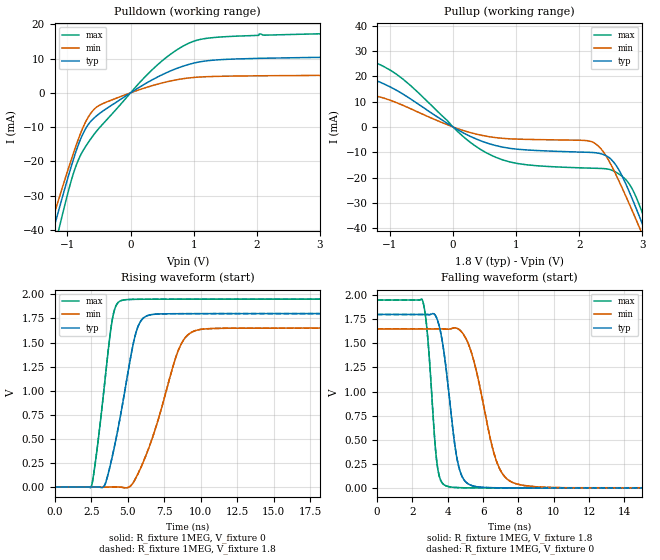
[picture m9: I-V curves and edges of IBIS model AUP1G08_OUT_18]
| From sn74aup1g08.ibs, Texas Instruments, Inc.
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[Model]   AUP1G08_OUT_18
Model_type  Output
Vref =   0
Rref =   1E6
Cref =   30p
Vmeas =   0.9
| variable   typ   min   max
C_comp   2.94pF   2.10pF   4.16pF
| C_pullup   3.20pF   2.10pF   4.16pF
| C_pulldown   2.68pF   2.30pF   3.20pF
[Temperature Range]   40   100   -40
| Ambient temperature   25   85   -40
[Voltage range]   1.8   1.65   1.95
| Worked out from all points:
|   slope of the pulldown table from 0 to 0.27 V, typ, clamps not added: 88.6 ohm
|   slope of the pullup table from 0 to 0.27 V, typ, clamps not added: 73.6 ohm
|   rising waveform, R_fixture 1MEG, V_fixture 0: 20-80 % time 1.31ns typ, 1.99ns min, 877ps max; typ from 0 V to 1.8 V
|   falling waveform, R_fixture 1MEG, V_fixture 1.8: 20-80 % time 712ps typ, 1.19ns min, 447ps max; typ from 1.8 V to 0 V
|   rising waveform, R_fixture 1MEG, V_fixture 1.8: 20-80 % time 1.31ns typ, 1.98ns min, 877ps max; typ from 0 V to 1.8 V
|   falling waveform, R_fixture 1MEG, V_fixture 0: 20-80 % time 712ps typ, 1.19ns min, 446ps max; typ from 1.8 V to 0 V
[Pulldown]
| AUP1G08_OUT_18
|   Voltage   I(typ)   I(min)   I(max)
-3.6V     -208.7mA   -190mA     -231.8mA
-1.27V    -43.18mA   -39.04mA   -50.16mA
-1.215V   -39.44mA   -35.69mA   -45.89mA
-1.125V   -33.4mA    -30.27mA   -38.98mA
-850mV    -16.32mA   -14.69mA   -20.63mA
-710mV    -10.41mA   -8.414mA   -15.6mA
-555mV    -6.973mA   -4.412mA   -11.55mA
360mV     3.96mA     2.185mA    7.039mA
705mV     6.927mA    3.722mA    12.18mA
1.03V     8.784mA    4.527mA    15.22mA
2.045V    10.05mA    4.967mA    17.16mA
7.2V      11.18mA    5.355mA    18.77mA
[Pullup]
| AUP1G08_OUT_18
|   Voltage   I(typ)   I(min)   I(max)
-3.6V     32.08mA    19.68mA    43.87mA
-3.16V    27.18mA    16.59mA    37.99mA
-2.12V    17.93mA    10.75mA    26.53mA
-1.525V   19.28mA    11.75mA    27.77mA
-1.155V   17.65mA    11.81mA    24.55mA
680mV     -7.373mA   -4.228mA   -12mA
2.185V    -10.05mA   -5.722mA   -16.26mA
2.485V    -12.35mA   -14.11mA   -16.81mA
2.725V    -21.82mA   -26.63mA   -20.47mA
2.94V     -34.57mA   -38.94mA   -30.09mA
3.085V    -43.77mA   -47.54mA   -39.78mA
7.2V      -335mA     -315.8mA   -357.8mA
[Ramp]
| AUP1G08_OUT_18
| variable   typ   min   max
dV/dt_r   1.08/1.32E-09   0.99/2.00E-09   1.17/8.81E-10
dV/dt_f   1.09/7.18E-10   1.00/1.20E-09   1.18/4.53E-10
R_load = 1MEG
[Rising Waveform]
| AUP1G08_OUT_18
R_fixture =   1MEG
C_fixture =   0
L_fixture =   0
V_fixture =   0
V_fixture_min = 0
V_fixture_max = 0
|   Time   V(typ)   V(min)   V(max)
0s        20.3nV     109.1nV    1.214nV
2.51ns    -41.4uV    2.109uV    10.3mV
3.365ns   8.497mV    -79.21uV   1.005V
3.91ns    297.3mV    803.3uV    1.71V
4.55ns    782.6mV    -1.29mV    1.935V
5.405ns   1.507V     54.03mV    1.948V
5.93ns    1.731V     214mV      1.949V
8.45ns    1.799V     1.413V     1.95V
9.585ns   1.799V     1.621V     1.95V
34.99ns   1.8V       1.65V      1.95V
[Falling Waveform]
| AUP1G08_OUT_18
R_fixture =   1MEG
C_fixture =   0
L_fixture =   0
V_fixture =   1.8
V_fixture_min = 1.65
V_fixture_max = 1.95
|   Time   V(typ)   V(min)   V(max)
0s        1.8V       1.65V      1.95V
2.57ns    1.8V       1.65V      1.944V
2.845ns   1.8V       1.65V      1.597V
3.395ns   1.751V     1.65V      243.1mV
3.975ns   1.126V     1.647V     16.31mV
4.465ns   362.5mV    1.659V     3.651mV
4.895ns   89.67mV    1.591V     1.071mV
6.745ns   1.096mV    283.4mV    101.7uV
7.885ns   255.2uV    41.61mV    91.85uV
34.99ns   149.3uV    244uV      90.05uV
[Rising Waveform]
| AUP1G08_OUT_18
R_fixture =   1MEG
C_fixture =   0
L_fixture =   0
V_fixture =   1.8
V_fixture_min = 1.65
V_fixture_max = 1.95
|   Time   V(typ)   V(min)   V(max)
0s        149.3uV    244uV      89.92uV
2.51ns    107.9uV    246uV      10.41mV
3.365ns   8.682mV    164.7uV    1.006V
3.91ns    297.8mV    1.047mV    1.71V
4.55ns    783.6mV    -1.046mV   1.935V
5.405ns   1.508V     54.52mV    1.948V
5.93ns    1.731V     214.8mV    1.949V
8.45ns    1.799V     1.414V     1.95V
9.58ns    1.799V     1.621V     1.95V
34.99ns   1.8V       1.65V      1.95V
[Falling Waveform]
| AUP1G08_OUT_18
R_fixture =   1MEG
C_fixture =   0
L_fixture =   0
V_fixture =   0
V_fixture_min = 0
V_fixture_max = 0
|   Time   V(typ)   V(min)   V(max)
0s        1.8V       1.65V      1.95V
2.57ns    1.8V       1.65V      1.944V
2.845ns   1.8V       1.65V      1.597V
3.395ns   1.751V     1.65V      242.8mV
3.975ns   1.126V     1.647V     16.2mV
4.465ns   362mV      1.659V     3.557mV
4.895ns   89.4mV     1.591V     979.3uV
6.745ns   941.9uV    282.8mV    11.76uV
7.885ns   105uV      41.17mV    1.918uV
34.99ns   21.4nV     91.24nV    133.5nV
